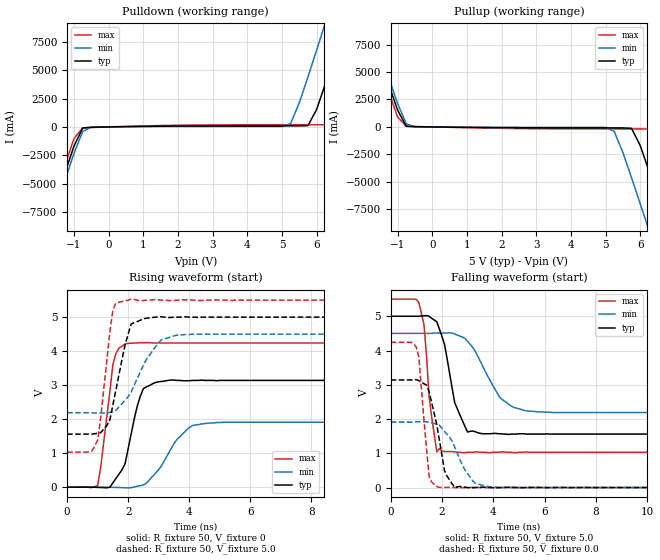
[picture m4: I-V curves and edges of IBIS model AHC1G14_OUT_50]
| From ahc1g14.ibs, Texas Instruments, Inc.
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|   Model AHC1G14_OUT_50
[Model]   AHC1G14_OUT_50
Model_type  Output
Polarity   Inverting
Vmeas = 2.50v
Cref = 15pf
| variable   typ   min   max
C_comp   3.12pf   2.34pf   3.90pf
[Temperature Range]   25   85   -40
[Voltage Range]   5.0   4.5   5.5
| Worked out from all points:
|   slope of the pulldown table from 0 to 0.75 V, typ, clamps not added: 18.8 ohm
|   slope of the pullup table from 0 to 0.75 V, typ, clamps not added: 25.3 ohm
|   rising waveform, R_fixture 50, V_fixture 0: 20-80 % time 478ps typ, 877ps min, 337ps max; typ from 0 V to 3.14 V
|   falling waveform, R_fixture 50, V_fixture 5.0: 20-80 % time 586ps typ, 1ns min, 310ps max; typ from 5 V to 1.56 V
|   rising waveform, R_fixture 50, V_fixture 5.0: 20-80 % time 478ps typ, 831ps min, 323ps max; typ from 1.56 V to 5 V
|   falling waveform, R_fixture 50, V_fixture 0.0: 20-80 % time 480ps typ, 798ps min, 289ps max; typ from 3.14 V to 0 V
[Pulldown]
|   Voltage   I(typ)   I(min)   I(max)
-5V       -40.9A     -41.4A     -40.3A
-1.75V    -8.76A     -9.39A     -8.09A
-1V       -1.69A     -2.33A     -1.02A
-750mV    -95.5mA    -395mA     -80.6mA
5.25V     93.4mA     298mA      192mA
5.75V     116mA      4.42A      192mA
6.25V     3.8A       9.19A      193mA
6.5V      6.17A      11.6A      931mA
6.75V     8.59A      14.1A      3.15A
7.25V     13.5A      19A        7.96A
7.5V      15.9A      21.4A      10.4A
10V       40.7A      46.2A      35.2A
[Pullup]
|   Voltage   I(typ)   I(min)   I(max)
-5V       40.7A      41.2A      40.1A
-2V       11A        11.6A      10.4A
-1.75V    8.59A      9.19A      7.96A
-1V       1.54A      2.14A      907mA
-750mV    63.6mA     284mA      62.5mA
5.25V     -84.4mA    -401mA     -178mA
5.75V     -130mA     -4.62A     -178mA
6.25V     -3.97A     -9.39A     -187mA
6.75V     -8.76A     -14.3A     -3.28A
7.25V     -13.6A     -19.2A     -8.09A
7.5V      -16.1A     -21.6A     -10.5A
10V       -40.9A     -46.4A     -35.3A
[Ramp]
| variable   typ   min   max
dV/dt_r   1.89E+00/4.48E-10   1.16E+00/7.78E-10   2.55E+00/3.01E-10
dV/dt_f   2.08E+00/5.39E-10   1.40E+00/1.03E-09   2.69E+00/3.03E-10
R_load = 50
[Rising Waveform]
R_fixture = 50
V_fixture = 0
|   Time   V(typ)   V(min)   V(max)
0s        0V         0V         0V
1ns       -6.14mV    320uV      48.5mV
1.5ns     127mV      -4.81mV    3.61V
1.9ns     692mV      -16.7mV    4.21V
2ns       1.13V      -19.9mV    4.23V
2.5ns     2.9V       66.2mV     4.25V
3.4ns     3.15V      1.12V      4.24V
4.1ns     3.14V      1.81V      4.24V
5.1ns     3.14V      1.91V      4.24V
25ns      3.14V      1.91V      4.24V
[Falling Waveform]
R_fixture = 50
V_fixture = 5.0
V_fixture_min = 4.5
V_fixture_max = 5.5
|   Time   V(typ)   V(min)   V(max)
0s        5V         4.5V       5.5V
1.1ns     5V         4.5V       5.4V
1.3ns     5.01V      4.5V       4.76V
1.5ns     5V         4.5V       2.65V
1.8ns     4.84V      4.51V      1.04V
2.5ns     2.47V      4.48V      1.04V
3ns       1.62V      4.27V      1.03V
4.3ns     1.57V      2.6V       1.04V
5.4ns     1.56V      2.23V      1.03V
25ns      1.56V      2.19V      1.03V
[Rising Waveform]
R_fixture = 50
V_fixture = 5.0
V_fixture_min = 4.5
V_fixture_max = 5.5
|   Time   V(typ)   V(min)   V(max)
0s        1.56V      2.19V      1.03V
800ps     1.56V      2.19V      1.05V
1ns       1.59V      2.18V      1.38V
1.4ns     1.97V      2.2V       4.56V
1.5ns     2.42V      2.21V      5.21V
1.9ns     4.19V      2.56V      5.48V
2.1ns     4.8V       2.8V       5.53V
3ns       5.02V      4.25V      5.51V
3.7ns     5V         4.48V      5.5V
25ns      5V         4.5V       5.5V
[Falling Waveform]
R_fixture = 50
V_fixture = 0.0
|   Time   V(typ)   V(min)   V(max)
0s        3.14V      1.91V      4.24V
1ns       3.15V      1.92V      4.1V
1.1ns     3.12V      1.92V      3.81V
1.5ns     2.8V       1.91V      322mV
1.9ns     1.39V      1.82V      7.43mV
2.1ns     492mV      1.64V      1.92mV
2.5ns     3.53mV     1.18V      642uV
3.2ns     -5.19mV    196mV      3.47mV
3.8ns     2.43mV     28.5mV     -3.1mV
25ns      0V         0V         0V
